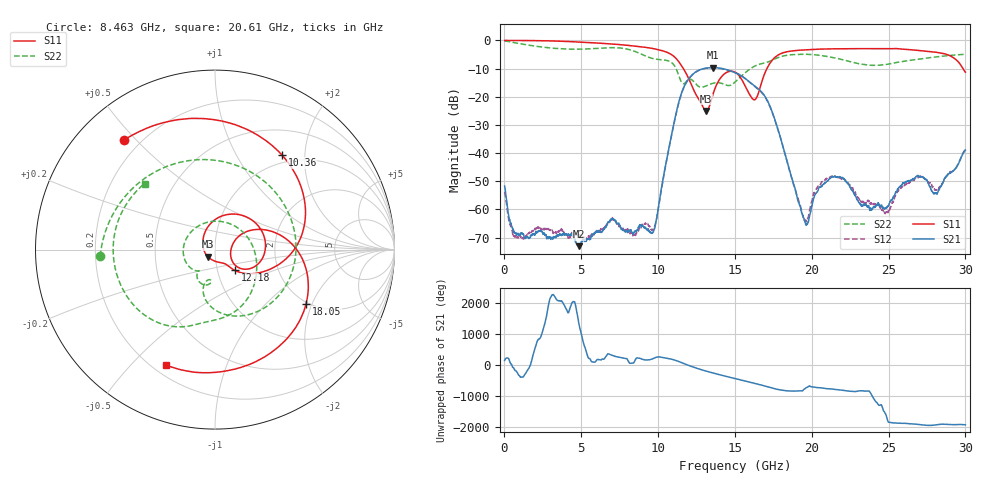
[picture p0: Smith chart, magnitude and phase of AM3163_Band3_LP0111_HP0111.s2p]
!Agilent Technologies,E8364B,MY43040894,A.07.50.67
!Agilent E8364B: A.07.50.67
!Date: Thursday, August 20, 2020 11:06:23
!Correction: S11(Full 2 Port(1,2))
!S21(Full 2 Port(1,2))
!S12(Full 2 Port(1,2))
!S22(Full 2 Port(1,2))
!S2P File: Measurements: S11, S21, S12, S22:
# Hz S  dB  R 50
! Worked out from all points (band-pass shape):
!   3201 points, 10 MHz to 30 GHz, reference 50 ohm
!   highest |S21| = -9.66 dB at 13.58 GHz (marker M1); lowest = -73.0 dB at 4.855 GHz (marker M2)
!   |S21| within 3 dB of the highest: 12.14 GHz to 15.44 GHz (3.297 GHz wide, 23.9 % of centre)
!   lowest |S11| = -25.0 dB at 13.13 GHz (marker M3), VSWR 1.12, Z = 46 - j3.63 ohm
!   |S11| at or under -10 dB: 11.64 GHz to 17.08 GHz (5.441 GHz wide, 37.9 % of centre); 29.83 GHz to end of sweep
!   |S22| runs from -16.6 to -0.2 dB; largest |S21 - S12| = 0.0059
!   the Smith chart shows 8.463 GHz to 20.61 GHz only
!   S11 on the Smith chart (normalised r, x): 8.463 GHz: 0.14, +0.46; 10.36 GHz: 0.87, +1.57; 12.18 GHz: 1.21, -0.29; 18.05 GHz: 1.94, -1.81; 20.61 GHz: 0.25, -0.63
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1e7  -0.04 -2.2  -51.70 153.9  -53.79 55.3  -0.20 -6.0
1.069022e9  -0.05 -29.0  -68.41 -31.6  -69.85 -143.4  -1.25 -83.5
2.381084e9  -0.13 -64.5  -67.67 -148.5  -66.99 -54.9  -2.33 -165.1
4.855259e9  -0.59 -129.4  -73.01 -135.1  -69.16 -81.2  -3.13 64.2
5.014581e9  -0.63 -133.6  -71.39 -91.6  -69.66 -73.2  -3.12 55.5
7.198228e9  -1.38 168.1  -63.89 -75.8  -64.43 -70.3  -2.60 -77.8
8.463431e9  -2.01 129.9  -67.76 118.6  -68.95 52.6  -3.87 -176.7
1.000979e10  -3.29 71.4  -59.63 -97.0  -59.74 -124.0  -6.79 27.4
1.035655e10  -3.80 54.8  -48.12 -117.0  -48.34 -117.0  -6.96 -9.4
1.218407e10  -15.93 -46.3  -12.41 -44.9  -12.49 -44.3  -13.97 -115.7
1.313062e10  -25.03 -135.4  -9.84 166.4  -9.89 166.7  -16.14 -130.3
1.358048e10  -19.02 119.8  -9.66 105.0  -9.74 105.3  -15.21 -149.0
1.5005e10  -11.27 -7.1  -11.45 -72.4  -11.41 -71.9  -14.82 35.0
1.628895e10  -21.05 -2.9  -16.21 133.2  -16.37 133.1  -9.13 -65.9
1.805086e10  -4.57 -30.9  -36.18 -86.7  -36.19 -83.8  -5.68 -129.6
1.952224e10  -3.37 -84.2  -63.72 -47.9  -63.87 103.5  -4.92 177.1
2.000958e10  -3.21 -97.7  -58.69 19.5  -57.03 10.7  -5.03 159.4
2.060938e10  -3.10 -113.0  -51.88 -14.3  -50.49 -17.6  -5.38 136.8
2.304607e10  -2.94 -168.9  -57.23 -112.3  -55.99 90.0  -8.27 23.4
2.500479e10  -2.99 144.9  -58.52 -39.6  -60.44 -6.6  -8.42 -81.4
2.734776e10  -3.81 79.7  -49.05 -132.0  -49.17 -127.9  -6.41 -173.4
3e10  -11.28 -20.7  -38.96 -122.0  -38.81 -124.2  -4.95 104.8
